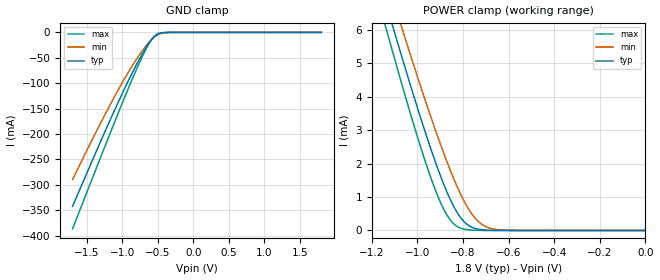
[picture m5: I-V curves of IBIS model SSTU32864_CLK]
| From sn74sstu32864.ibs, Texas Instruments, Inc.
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[Model]   SSTU32864_CLK
Model_type  Input
Vinl=1.125
Vinh=0.675
| variable   typ   min   max
C_comp   2.31pF   1.84pF   2.53pF
[Temperature Range]   40   85   0
| Ambient temperature   25   70   0
[Voltage range]   1.8   1.7   1.9
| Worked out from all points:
|   GND clamp passes 1 mA (typ) near -0.44 V on its own axis
|   POWER clamp passes 1 mA (typ) near -0.86 V on its own axis
[GND Clamp]
| SSTU32864_CLK
|   Voltage   I(typ)   I(min)   I(max)
-1.7V     -342.1mA   -289.5mA   -386.2mA
-1.285V   -208.1mA   -172.9mA   -238.4mA
-1.115V   -154.9mA   -127.8mA   -178.6mA
-970mV    -111.1mA   -91.47mA   -128.6mA
-810mV    -65.85mA   -54.8mA    -75.73mA
-680mV    -33.18mA   -28.91mA   -36.39mA
-600mV    -16.47mA   -15.74mA   -16.47mA
-530mV    -6.263mA   -7.094mA   -5.307mA
-455mV    -1.321mA   -1.982mA   -848uA
-335mV    -44.15uA   -113.6uA   -15.67uA
1.8V      1.13nA     9.072nA    128pA
[POWER Clamp]
| SSTU32864_CLK
|   Voltage   I(typ)   I(min)   I(max)
-1.7V     20.54mA    20.56mA    20.57mA
-1.14V    6.837mA    7.627mA    6.099mA
-1.1V     5.907mA    6.744mA    5.124mA
-1.06V    4.993mA    5.872mA    4.169mA
-980mV    3.235mA    4.179mA    2.363mA
-915mV    1.926mA    2.879mA    1.097mA
-865mV    1.061mA    1.956mA    400.2uA
-820mV    474.7uA    1.221mA    98.68uA
-785mV    198uA      747uA      26uA
-745mV    57.1uA     352.4uA    5.154uA
-670mV    4.139uA    49.18uA    235.7nA
-14.28fV  1.13nA     8.645nA    145.4pA
